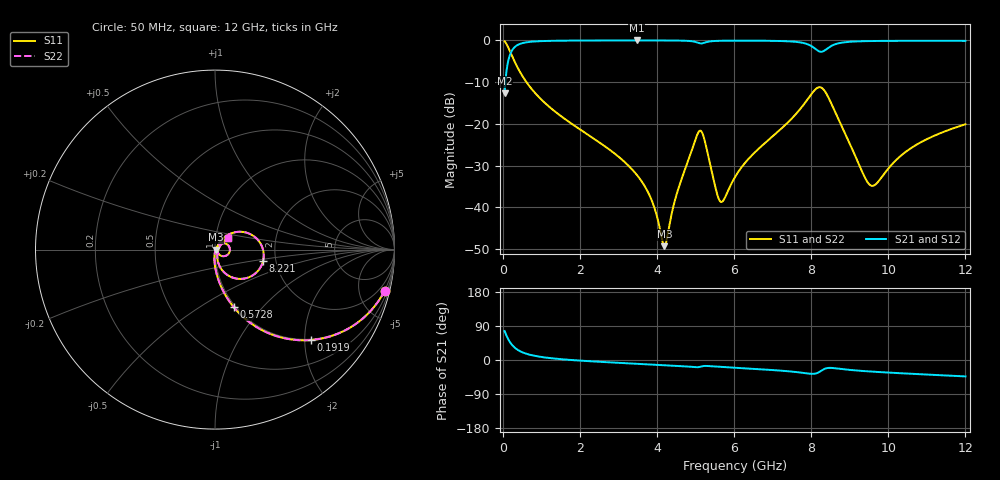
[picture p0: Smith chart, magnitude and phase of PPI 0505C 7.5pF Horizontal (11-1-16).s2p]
# MHz S MA R 50
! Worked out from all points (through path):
!   1601 points, 50 MHz to 12 GHz, reference 50 ohm
!   highest |S21| = -0.02 dB at 3.471 GHz (marker M1); lowest = -12.7 dB at 50 MHz (marker M2)
!   group delay of S21, straight-line fit = 13.5 ps
!   lowest |S11| = -49.3 dB at 4.195 GHz (marker M3), VSWR 1.01, Z = 50.3 - j0.112 ohm
!   |S11| at or under -10 dB: 616.3 MHz to end of sweep
!   |S22| runs from -49.3 to -0.2 dB; largest |S21 - S12| = 0
!   S11 on the Smith chart (normalised r, x): 50 MHz: 0.98, -8.25; 191.9 MHz: 0.98, -2.15; 572.8 MHz: 0.98, -0.71; 8.221 GHz: 1.71, -0.24; 12 GHz: 1.15, +0.15
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50  0.9725 -13.6  0.2329 76.4  0.2329 76.4  0.9725 -13.6
191.9062  0.7356 -43.2  0.677 46.7  0.677 46.7  0.7356 -43.2
348.75  0.5116 -60.3  0.8585 29.6  0.8585 29.6  0.5116 -60.3
572.8125  0.3382 -71.9  0.9401 17.9  0.9401 17.9  0.3382 -71.9
2044.156  0.08355 -90.7  0.9947 -1.9  0.9947 -1.9  0.08355 -90.7
3470.688  0.02481 -94.5  0.9972 -9.9  0.9972 -9.9  0.02481 -94.5
3814.25  0.01379 -90.6  0.997 -11.6  0.997 -11.6  0.01379 -90.6
4038.312  0.0067 -76.0  0.9967 -12.8  0.9967 -12.8  0.0067 -76.0
4195.156  0.00344 -18.8  0.9963 -13.6  0.9963 -13.6  0.00344 -18.8
4546.188  0.01624 53.7  0.9939 -15.6  0.9939 -15.6  0.01624 53.7
5091.406  0.08141 9.2  0.927 -18.6  0.927 -18.6  0.08141 9.2
5218.375  0.06836 -30.7  0.9334 -15.9  0.9334 -15.9  0.06836 -30.7
5636.625  0.01187 -10.2  0.9879 -18.3  0.9879 -18.3  0.01187 -10.2
6025  0.02311 50.3  0.9918 -20.7  0.9918 -20.7  0.02311 50.3
7414.188  0.1061 49.2  0.9737 -29.8  0.9737 -29.8  0.1061 49.2
8019.156  0.2315 18.1  0.8475 -36.5  0.8475 -36.5  0.2315 18.1
8220.812  0.2751 -13.5  0.7336 -31.0  0.7336 -31.0  0.2751 -13.5
8676.406  0.1225 -70.6  0.9137 -22.4  0.9137 -22.4  0.1225 -70.6
9490.5  0.01928 -34.8  0.9802 -30.1  0.9802 -30.1  0.01928 -34.8
10013.31  0.02969 30.6  0.986 -33.3  0.986 -33.3  0.02969 30.6
10782.59  0.05813 43.0  0.988 -37.3  0.988 -37.3  0.05813 43.0
12000  0.09899 42.0  0.9863 -43.3  0.9863 -43.3  0.09899 42.0
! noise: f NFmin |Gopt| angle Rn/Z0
50  0.0004629  0.8915  1.848  0.0009285
1372  0.004369  0.6986  4.995  0.002829
2701  0.007257  0.653  9.062  0.003956
4031  0.01111  0.6614  13.1  0.006196
5360  0.04036  0.8619  17.33  0.06124
6682  0.02338  0.7265  21.33  0.01643
8012  0.1081  0.9217  25.58  0.2907
9341  0.04547  0.7988  29.72  0.04377
1.067e+04  0.03236  0.6984  33.51  0.01929
1.2e+04  0.03086  0.6572  37.14  0.01551
